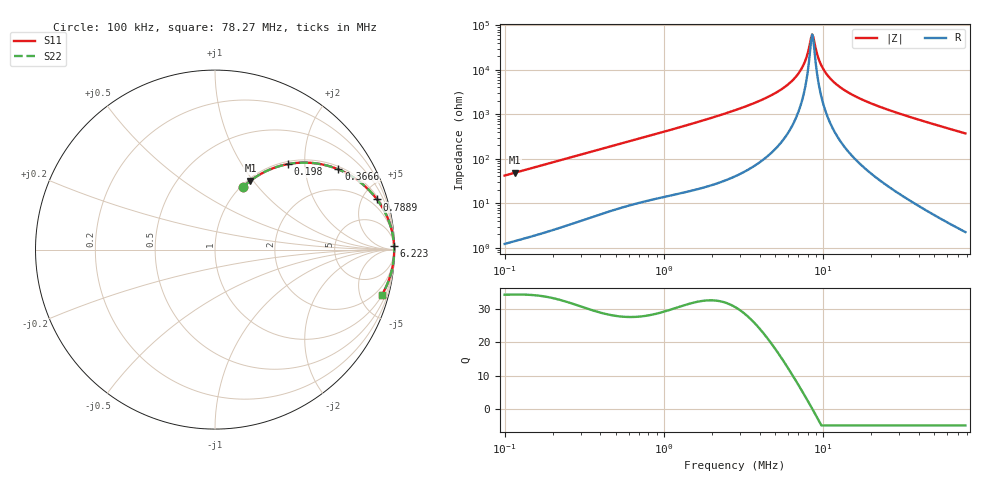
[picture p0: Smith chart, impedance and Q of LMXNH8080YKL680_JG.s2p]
! LMXNH8080YKL680_JG  S-PARAMETER MODEL  ( General Type )
! Model Generated by TAIYO YUDEN Corporation (https://www.yuden.co.jp/en/)
! Version 1.0
! TAIYO YUDEN Control No. 200915NI43SB-FBB
! Copyright(c) 2020 TAIYO YUDEN CO.,LTD. All Rights Reserved.
! Product Description (link to TY-COMPAS)
! https://ds.yuden.co.jp/TYCOMPAS/or/detail?pn=LMXNH8080YKL680MJG&u=M
! Products Name : Inductors
! Characteristics :
!  Inductance : 68 uH , SRF(min) : 7.0 MHz , DC Resistance(max) : 0.273 Ohm
!  Rated Current : Saturation :1300 mA , Temp Rise : 1200 mA (40 degC)
!  Case Size : 8.0 x 8.0 / 0.315 x 0.315 [mm/inch] , Thickness : 4 / 0.157 [mm/inch]
!  (Conditions: Temperature = 25 degC , DC Bias Current/Voltage = 0A / 0V)
! External Node Assignments :
!  1  o---GGG---o  2
! GND o---------o GND
! Frequency Range : 0.1MHz  -  78.268192MHz  [ 402 STEP ]
# MHz S RI R 50
! Freq[MHz].  S11 Real  S11 Imag  S21 Real  S21 Imag  S12 Real  S12 Imag  S22 Real  S22 Imag
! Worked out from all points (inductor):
!   401 points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, 100 kHz to 78.27 MHz, reference 50 ohm
!   read as one part in series: L = 66.3 uH near 103.4 kHz
!   highest Q = 34.4 at 116.2 kHz (marker M1), where L = 66.4 uH
!   self-resonance near 8.54 MHz
!   S11 on the Smith chart (normalised r, x): 100 kHz: 1.02, +0.84; 198 kHz: 1.05, +1.64; 366.6 kHz: 1.10, +3.00; 788.9 kHz: 1.23, +6.37; 6.223 MHz: open; 78.27 MHz: 1.04, -7.42
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0.1  0.1562 0.3488  0.8438 -0.3488  0.8438 -0.3488  0.1562 0.3488
0.116173  0.1974 0.3838  0.8026 -0.3838  0.8026 -0.3838  0.1974 0.3838
0.197967  0.4049 0.4761  0.5951 -0.4761  0.5951 -0.4761  0.4049 0.4761
0.305264  0.6085 0.4721  0.3915 -0.4721  0.3915 -0.4721  0.6085 0.4721
0.366648  0.6873 0.4469  0.3127 -0.4469  0.3127 -0.4469  0.6873 0.4469
0.788881  0.9023 0.2797  0.0977 -0.2797  0.0977 -0.2797  0.9023 0.2797
0.931861  0.9267 0.2439  0.0733 -0.2439  0.0733 -0.2439  0.9267 0.2439
2.844635  0.9912 0.0786  0.00884 -0.0786  0.00884 -0.0786  0.9912 0.0786
4.611174  0.9966 0.039  0.00344 -0.039  0.00344 -0.039  0.9966 0.039
6.223331  0.9979 0.0192  0.00209 -0.0192  0.00209 -0.0192  0.9979 0.0192
6.877438  0.9982 0.0131  0.00185 -0.0131  0.00185 -0.0131  0.9982 0.0131
7.474747  0.9983 0.00803  0.00171 -0.00803  0.00171 -0.00803  0.9983 0.00803
7.857753  0.9983 0.00504  0.00165 -0.00504  0.00165 -0.00504  0.9983 0.00504
8.399128  0.9984 0.00108  0.00161 -0.00108  0.00161 -0.00108  0.9984 0.00108
8.540203  0.9984 9.07e-05  0.00161 -9.07e-05  0.00161 -9.07e-05  0.9984 9.07e-05
8.8295  0.9984 -0.00189  0.0016 0.00189  0.0016 0.00189  0.9984 -0.00189
9.281924  0.9984 -0.00486  0.00161 0.00486  0.00161 0.00486  0.9984 -0.00486
9.921421  0.9983 -0.00885  0.00165 0.00885  0.00165 0.00885  0.9983 -0.00885
11.71962  0.9981 -0.019  0.00191 0.019  0.00191 0.019  0.9981 -0.019
15.81703  0.997 -0.0388  0.00303 0.0388  0.00303 0.0388  0.997 -0.0388
26.07016  0.992 -0.0803  0.00801 0.0803  0.00801 0.0803  0.992 -0.0803
78.26819  0.931 -0.2505  0.069 0.2505  0.069 0.2505  0.931 -0.2505
